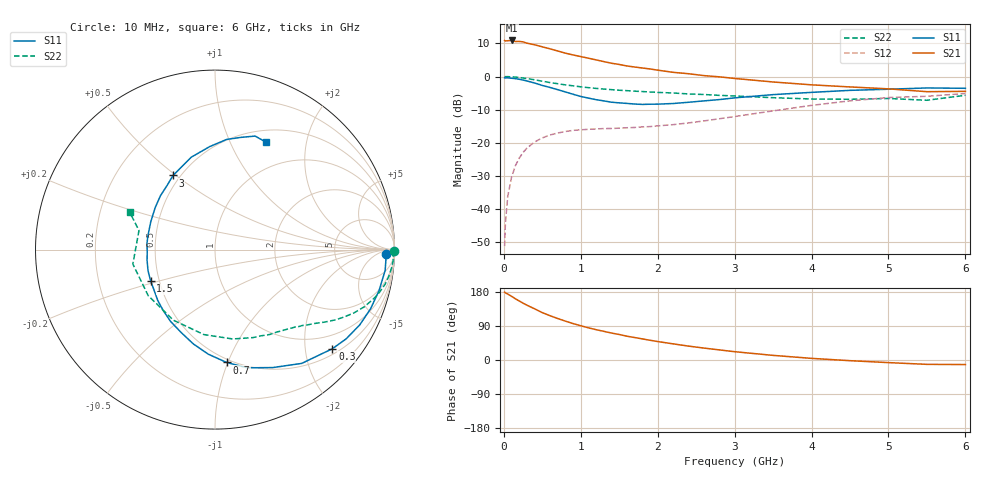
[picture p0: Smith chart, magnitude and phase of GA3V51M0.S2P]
! Infineon Technologies  Discrete & RF Semiconductors
! BF775
! Si NPN RF Bipolar Junction Transistor in SOT23
! VCE = 3.5 V  IC = 1 mA
! Common Emitter S-Parameters:  May  1996
# GHz  S  MA  R  50
!  f  S11  S21  S12  S22
! GHz  MAG  ANG  MAG  ANG  MAG  ANG  MAG  ANG
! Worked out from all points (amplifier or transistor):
!   36 points, 10 MHz to 6 GHz, reference 50 ohm
!   highest |S21| = 10.9 dB at 100 MHz (marker M1)
!   |S21| within 3 dB of that: start of sweep to 671.5 MHz
!   unconditionally stable (mu >= 1): 1.414 GHz to 4.142 GHz; 5.056 GHz to end of sweep
!   at 250 MHz: K = 0.21, MSG = 16.7 dB, |S12| = -23.0 dB
!   at 1.4 GHz: K = 0.99, MSG = 9.9 dB, |S12| = -15.7 dB
!   at 6 GHz: K = 1.03, MAG = -0.7 dB, |S12| = -5.2 dB
!   S11 on the Smith chart (normalised r, x): 10 MHz: 33, -19; 300 MHz: 0.63, -2.60; 700 MHz: 0.47, -0.99; 1.5 GHz: 0.45, -0.19; 3 GHz: 0.46, +0.49; 6 GHz: 0.64, +1.37
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0.01  0.9553 -1.5  3.506 179.2  0.0027 92.5  0.9999 -0.6
0.02  0.9541 -2.8  3.447 177.4  0.0059 88.5  0.9925 -1.2
0.05  0.9551 -7.0  3.477 174.0  0.0151 85.2  0.9956 -3.0
0.1  0.942 -14.0  3.513 168.2  0.0299 81.5  0.9888 -6.0
0.15  0.9275 -20.8  3.388 161.5  0.0445 76.9  0.9791 -8.9
0.2  0.909 -27.5  3.397 155.8  0.058 72.9  0.9666 -11.6
0.25  0.884 -34.2  3.345 150.0  0.0708 68.7  0.9484 -14.3
0.3  0.8559 -40.2  3.199 144.6  0.0824 65.4  0.93 -16.7
0.4  0.7971 -52.7  3.022 135.1  0.1022 58.6  0.8916 -20.9
0.5  0.7319 -63.9  2.813 125.0  0.1177 53.0  0.8494 -24.6
0.7  0.6322 -84.1  2.434 109.5  0.1393 44.4  0.7776 -30.2
0.9  0.5389 -103.0  2.119 96.1  0.1529 38.6  0.7222 -34.2
1.1  0.4706 -121.7  1.892 84.9  0.1587 35.1  0.6776 -37.8
1.5  0.3991 -153.8  1.521 67.3  0.1652 33.2  0.6197 -44.2
1.9  0.3806 174.6  1.301 52.1  0.1744 35.6  0.583 -51.2
2.2  0.39 156.6  1.157 42.6  0.1866 38.1  0.5628 -57.2
3  0.4747 119.5  0.934 21.9  0.2475 42.9  0.5075 -78.8
3.5  0.5316 104.4  0.826 12.2  0.3016 41.3  0.4776 -97.4
4.5  0.617 84.0  0.695 -1.8  0.4278 30.2  0.452 -145.4
5  0.6417 77.0  0.65 -6.9  0.48 22.2  0.4647 -170.0
5.5  0.6709 70.5  0.589 -11.5  0.5017 13.1  0.4367 165.9
6  0.6627 64.8  0.596 -12.0  0.5523 8.3  0.5194 156.3
